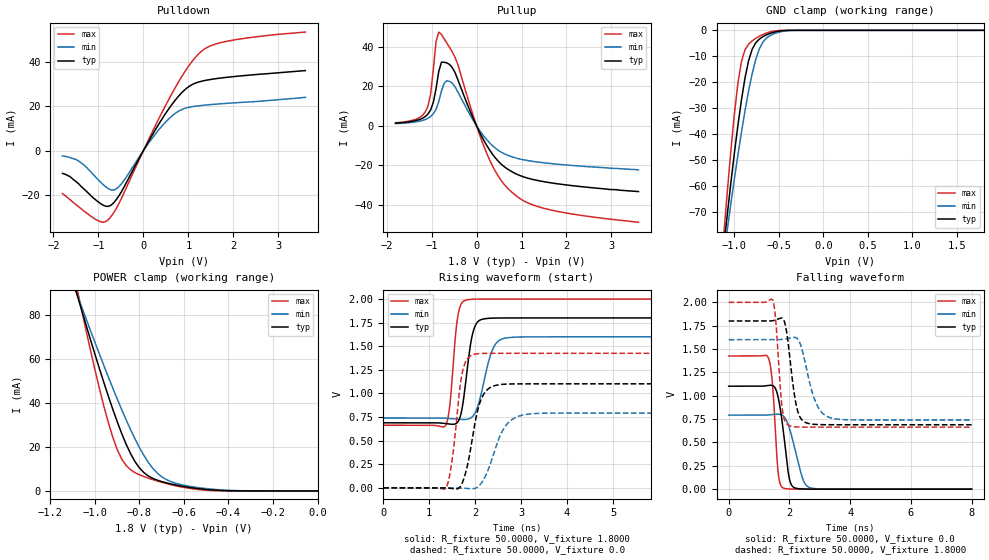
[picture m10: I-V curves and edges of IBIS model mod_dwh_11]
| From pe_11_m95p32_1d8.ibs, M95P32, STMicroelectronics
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|   Model mod_dwh_11
[Model]   mod_dwh_11
Model_type I/O
Polarity   Non-Inverting
Enable   Active-High
Vinl   =   0.540V
Vinh   =   1.260V
Vmeas  =   0.900V
Cref   =   30.0pF
C_comp   1.630pF   1.607pF   1.683pF
[Model Spec]
Vinl   0.540V  0.480V  0.600V  | <- for Vcc = 1.8V, 1.6V, 2.0V
Vinh   1.260V  1.120V  1.400V  | <- for Vcc = 1.8V, 1.6V, 2.0V
Vmeas  0.900V  0.800V  1.000V  | <- for Vcc = 1.8V, 1.6V, 2.0V
[Temperature Range]  25.0000   0.1050k   -40.0000
[Voltage Range]   1.8000V   1.6000V   2.0000V
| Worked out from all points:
|   slope of the pulldown table from 0 to 0.27 V, typ, clamps not added: 28.4 ohm
|   slope of the pullup table from 0 to 0.27 V, typ, clamps not added: 23.5 ohm
|   GND clamp passes 1 mA (typ) near -0.58 V on its own axis
|   POWER clamp passes 1 mA (typ) near -0.53 V on its own axis
|   rising waveform, R_fixture 50.0000, V_fixture 1.8000: 20-80 % time 182ps typ, 262ps min, 138ps max; typ from 0.689 V to 1.8 V
|   rising waveform, R_fixture 50.0000, V_fixture 0.0: 20-80 % time 265ps typ, 376ps min, 194ps max; typ from 0 V to 1.1 V
|   falling waveform, R_fixture 50.0000, V_fixture 0.0: 20-80 % time 254ps typ, 375ps min, 162ps max; typ from 1.1 V to 0 V
|   falling waveform, R_fixture 50.0000, V_fixture 1.8000: 20-80 % time 264ps typ, 425ps min, 171ps max; typ from 1.8 V to 0.689 V
[Pulldown]
|Voltage   I(typ)   I(min)   I(max)
-1.8V     -10.24mA   -2.4mA     -19.3mA
-1.38V    -16.2mA    -5.5mA     -26.2mA
-1.02V    -22.81mA   -12.77mA   -31.38mA
-840mV    -25mA      -16.21mA   -31.94mA
-660mV    -23.45mA   -17.74mA   -27.95mA
-540mV    -20.2mA    -16.11mA   -23.67mA
240mV     8.511mA    6.772mA    10.14mA
660mV     21.45mA    16mA       26.6mA
960mV     28.04mA    19.23mA    36.67mA
1.26V     31.03mA    20.24mA    44.14mA
1.86V     32.97mA    21.27mA    49.19mA
3.6V      36mA       23.99mA    53.3mA
[Pullup]
|Voltage   I(typ)   I(min)   I(max)
-1.8V     1.33mA     1.08mA     1.52mA
-1.14V    4.66mA     3.15mA     6.95mA
-1.02V    8.045mA    4.677mA    16.05mA
-900mV    18.77mA    8.355mA    42.54mA
-840mV    27.4mA     12.2mA     47.42mA
-780mV    32.19mA    17.56mA    46.22mA
-720mV    32.13mA    21.49mA    44.06mA
-540mV    29.45mA    21.6mA     37.4mA
240mV     -10.43mA   -7.367mA   -14.65mA
720mV     -22.36mA   -15.17mA   -32.25mA
1.56V     -28.54mA   -18.9mA    -42.13mA
3.6V      -33.3mA    -22.3mA    -48.8mA
[GND_clamp]
|Voltage   I(typ)   I(min)   I(max)
-1.8V     -319.7mA   -274.4mA   -407.3mA
-1.12V    -83.64mA   -87.01mA   -79.32mA
-1.08V    -71.08mA   -76.85mA   -62.45mA
-1V       -47.38mA   -57.28mA   -32.33mA
-960mV    -36.55mA   -47.99mA   -20.38mA
-920mV    -26.73mA   -39.15mA   -11.92mA
-840mV    -11.67mA   -23.32mA   -5.34mA
-760mV    -4.801mA   -11.23mA   -3.081mA
-720mV    -3.384mA   -7.183mA   -2.279mA
-640mV    -1.748mA   -2.99mA    -1.048mA
-440mV    -85.93uA   -314uA     -8.035uA
1.8V      367pA      1.678uA    95.55pA
[POWER_clamp]
|Voltage   I(typ)   I(min)   I(max)
-1.8V     354.3mA    299.2mA    462.7mA
-1.08V    89.41mA    89.52mA    92.12mA
-1.06V    82.53mA    84.01mA    82.65mA
-980mV    55.86mA    62.44mA    46.9mA
-920mV    37.35mA    46.96mA    24.63mA
-880mV    26.31mA    37.17mA    14.66mA
-840mV    17.07mA    28.03mA    9.669mA
-800mV    10.51mA    19.82mA    7.37mA
-740mV    5.731mA    10.32mA    5.151mA
-640mV    2.77mA     3.598mA    2.408mA
-420mV    154.7uA    391.9uA    29.01uA
0V        367pA      12.25nA    169pA
[Ramp]
| variable   typ   min   max
dV/dt_r   0.6613/0.3068n   0.4755/0.4810n   0.8553/0.2231n
dV/dt_f   0.6665/0.3066n   0.5161/0.5714n   0.8018/0.1879n
R_load = 50.0000
[Rising Waveform]
R_fixture= 50.0000
V_fixture= 1.8000
V_fixture_min= 1.6000
V_fixture_max= 2.0000
|time   V(typ)   V(min)   V(max)
0s        689.2mV    739.9mV    663.6mV
1.35ns    681.8mV    738.3mV    657.1mV
1.45ns    675.4mV    734.6mV    889.9mV
1.61ns    691.8mV    727.9mV    1.785V
1.79ns    1.109V     724.4mV    1.988V
1.91ns    1.555V     742.5mV    1.998V
2.01ns    1.728V     806mV      1.999V
2.35ns    1.798V     1.432V     2V
2.61ns    1.8V       1.582V     2V
8ns       1.8V       1.6V       2V
[Rising Waveform]
R_fixture= 50.0000
V_fixture= 0.0
V_fixture_min= 0.0
V_fixture_max= 0.0
|time   V(typ)   V(min)   V(max)
0s        2.875nV    388.8nV    438.6pV
1.37ns    -598.4uV   604.7uV    5.172mV
1.51ns    -7.96mV    432.9uV    338.2mV
1.71ns    44.42mV    -2.328mV   1.202V
1.95ns    562.2mV    -9.196mV   1.411V
2.09ns    886.2mV    25.06mV    1.422V
2.25ns    1.034V     154.5mV    1.425V
2.61ns    1.097V     619mV      1.425V
2.99ns    1.102V     765.7mV    1.425V
8ns       1.102V     792.6mV    1.425V
[Falling Waveform]
R_fixture= 50.0000
V_fixture= 0.0
V_fixture_min= 0.0
V_fixture_max= 0.0
|time   V(typ)   V(min)   V(max)
0s        1.102V     792.6mV    1.425V
1.32ns    1.111V     794.6mV    1.395V
1.44ns    1.11V      798.4mV    1.137V
1.62ns    998.1mV    802.9mV    209.4mV
1.78ns    674.3mV    788.4mV    14.85mV
1.94ns    226.8mV    707.4mV    3.183mV
2.04ns    65.62mV    608.6mV    1.295mV
2.42ns    2.5mV      128.7mV    43.23uV
2.66ns    519.1uV    17.59mV    6.735uV
8ns       691.5nV    993.2nV    774.6nV
[Falling Waveform]
R_fixture= 50.0000
V_fixture= 1.8000
V_fixture_min= 1.6000
V_fixture_max= 2.0000
|time   V(typ)   V(min)   V(max)
0s        1.8V       1.6V       2V
1.45ns    1.803V     1.599V     2.023V
1.55ns    1.812V     1.6V       1.807V
1.77ns    1.829V     1.604V     844.5mV
1.99ns    1.478V     1.616V     681.6mV
2.25ns    862.5mV    1.614V     665.7mV
2.55ns    711.1mV    1.307V     663.8mV
2.89ns    692.2mV    913.6mV    663.6mV
3.33ns    689.5mV    766.4mV    663.6mV
8ns       689.2mV    739.9mV    663.6mV
